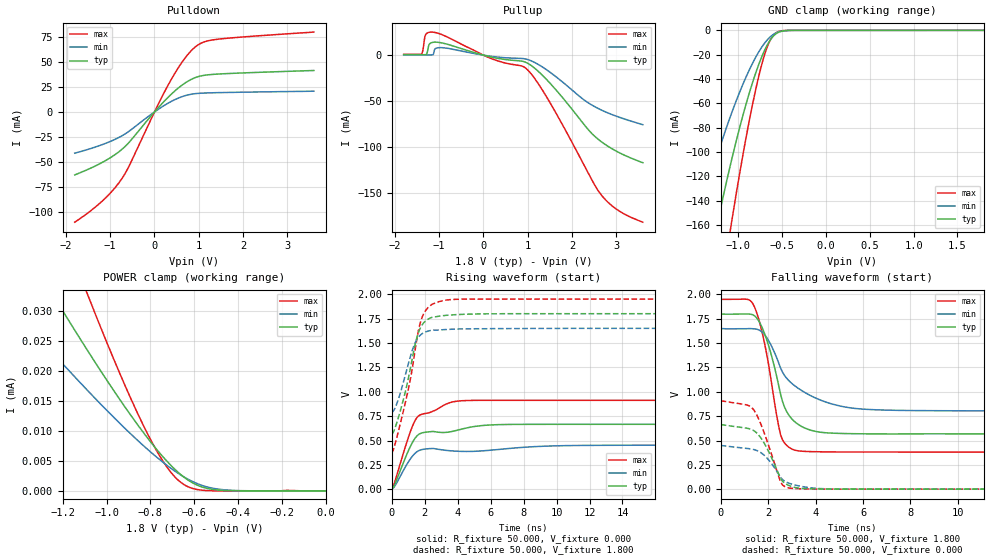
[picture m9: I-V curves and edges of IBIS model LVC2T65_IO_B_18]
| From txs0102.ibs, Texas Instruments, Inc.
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[Model]   LVC2T65_IO_B_18
Model_type  I/O
Vinl=0.15
Vinh=1.25
Enable   Active-High
Vref =   1.8V
Rref =   1000000
Cref =   15p
Vmeas =   0.9
| variable   typ   min   max
C_comp   7.28pF   6.26pF   7.93pF
| C_pullup   7.12pF   6.34pF   8.49pF
| C_pulldown   8.27pF   6.85pF   9.45pF
| C_tri-state   7.28pF   6.26pF   7.93pF
[Temperature Range]   40   100   -40
| Ambient temperature   25   85   -40
[Voltage range]   1.8   1.65   1.95
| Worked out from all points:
|   slope of the pulldown table from 0 to 0.27 V, typ, clamps not added: 20.8 ohm
|   slope of the pullup table from 0 to 0.27 V, typ, clamps not added: 89.3 ohm
|   GND clamp passes 1 mA (typ) near -0.52 V on its own axis
|   rising waveform, R_fixture 50.000, V_fixture 0.000: 20-80 % time 1.07ns typ, 979ps min, 1.12ns max; typ from 0.003 V to 0.665 V
|   falling waveform, R_fixture 50.000, V_fixture 1.800: 20-80 % time 837ps typ, 1.65ns min, 689ps max; typ from 1.8 V to 0.566 V
|   rising waveform, R_fixture 50.000, V_fixture 1.800: 20-80 % time 988ps typ, 887ps min, 1.09ns max; typ from 0.566 V to 1.8 V
|   falling waveform, R_fixture 50.000, V_fixture 0.000: 20-80 % time 803ps typ, 873ps min, 786ps max; typ from 0.665 V to 0.002 V
[GND Clamp]
| LVC2T65_IO_B_18
|   Voltage   I(typ)   I(min)   I(max)
-1.8V     -375.4mA   -251.7mA   -534.8mA
-1.505V   -256mA     -168.2mA   -372.2mA
-1.455V   -236.9mA   -155.1mA   -345.5mA
-1.245V   -161.1mA   -104mA     -237.8mA
-1.085V   -109.4mA   -69.9mA    -161.9mA
-1.065V   -103.3mA   -65.96mA   -152.9mA
-910mV    -60.44mA   -38.25mA   -87.94mA
-790mV    -32.88mA   -20.73mA   -45.28mA
-690mV    -15.04mA   -9.675mA   -17.94mA
-595mV    -4.452mA   -3.158mA   -3.768mA
-435mV    -133uA     -140.9uA   -36.64uA
1.8V      221.9pA    1.807nA    42.15pA
[POWER Clamp]
| LVC2T65_IO_B_18
|   Voltage   I(typ)   I(min)   I(max)
-1.8V     67.65uA    46.37uA    105uA
-1.475V   46.79uA    32.42uA    70.89uA
-1.245V   32.66uA    22.95uA    47.81uA
-1.09V    23.55uA    16.85uA    33uA
-1.045V   21uA       15.13uA    28.85uA
-900mV    13.13uA    9.844uA    16.23uA
-820mV    9.138uA    7.145uA    10.01uA
-740mV    5.561uA    4.691uA    4.787uA
-660mV    2.669uA    2.614uA    1.382uA
-585mV    936.6nA    1.193uA    222.3nA
-495mV    158.1nA    315.9nA    13.45nA
0V        0A         0A         0A
[Pulldown]
| LVC2T65_IO_B_18
|   Voltage   I(typ)   I(min)   I(max)
-1.8V     -62.77mA   -41.14mA   -109.8mA
-1.16V    -49.87mA   -32.31mA   -88.04mA
-950mV    -44.35mA   -28.57mA   -78.6mA
-750mV    -37.89mA   -24.23mA   -67.42mA
-575mV    -30.5mA    -19.34mA   -54.13mA
35mV      1.607mA    980.9uA    2.933mA
355mV     16.51mA    9.772mA    30.32mA
665mV     27.92mA    15.73mA    52.05mA
940mV     34.37mA    18.2mA     65.23mA
1.13V     36.41mA    18.73mA    69.74mA
1.455V    37.68mA    19.14mA    72.43mA
3.6V      41.17mA    20.55mA    79.4mA
[Pullup]
| LVC2T65_IO_B_18
|   Voltage   I(typ)   I(min)   I(max)
-1.8V     498.7uA    245.1uA    961uA
-1.395V   487.4uA    239.5uA    1.376mA
-1.305V   513.2uA    237.4uA    22.18mA
-1.225V   11.59mA    235.4uA    24.83mA
-1.135V   13.99mA    587.7uA    24.97mA
-1.08V    14.15mA    7.254mA    24.52mA
-925mV    13.2mA     8.13mA     22.11mA
150mV     -1.808mA   -1.097mA   -3.195mA
925mV     -7.183mA   -3.91mA    -13.08mA
1.415V    -25.86mA   -15.49mA   -44.39mA
2.675V    -94.48mA   -59.88mA   -152.7mA
3.6V      -116.9mA   -75.54mA   -181.5mA
[Ramp]
| LVC2T65_IO_B_18
| variable   typ   min   max
dV/dt_r   0.43/1.07E-09   0.29/9.87E-10   0.58/1.13E-09
dV/dt_f   0.73/8.35E-10   0.49/1.65E-09   0.94/6.86E-10
R_load = 50
[Rising Waveform]
R_fixture = 50.000
V_fixture = 0.000
V_fixture_min = 0.000
V_fixture_max = 0.000
C_fixture = 0.000
L_fixture = 0.000
|  time   V(typ)   V(min)   V(max)
0s        2.79mV     2.781mV    2.705mV
168ps     44.99mV    29.35mV    68.73mV
1.176ns   455.6mV    323.4mV    612.8mV
1.596ns   558.2mV    393.1mV    748.4mV
2.52ns    593.8mV    419.6mV    803.2mV
3.528ns   589.7mV    396.4mV    888.7mV
4.956ns   643.1mV    390.2mV    912.1mV
9.324ns   667mV      443.2mV    912.8mV
14.95ns   667mV      452.7mV    912.7mV
419.9ns   665.1mV    451.2mV    909mV
[Falling Waveform]
R_fixture = 50.000
V_fixture = 1.800
V_fixture_min = 1.650
V_fixture_max = 1.950
C_fixture = 0.000
L_fixture = 0.000
|  time   V(typ)   V(min)   V(max)
0s        1.799V     1.649V     1.95V
1.428ns   1.778V     1.645V     1.868V
1.932ns   1.539V     1.558V     1.395V
2.436ns   1.074V     1.301V     657.8mV
2.688ns   845mV      1.168V     475.5mV
3.276ns   664.2mV    1.034V     394.6mV
4.2ns     585.7mV    915.4mV    385mV
6.048ns   569.2mV    821.5mV    382.6mV
11.09ns   568mV      804.8mV    382.4mV
419.9ns   566.4mV    790.8mV    381.8mV
[Rising Waveform]
R_fixture = 50.000
V_fixture = 1.800
V_fixture_min = 1.650
V_fixture_max = 1.950
C_fixture = 0.000
L_fixture = 0.000
|  time   V(typ)   V(min)   V(max)
0s        566mV      790.1mV    371mV
336ps     699.1mV    891.2mV    551.2mV
924ps     1.072V     1.234V     961.8mV
1.176ns   1.28V      1.386V     1.169V
1.512ns   1.548V     1.533V     1.529V
1.68ns    1.634V     1.571V     1.674V
1.848ns   1.687V     1.596V     1.766V
2.436ns   1.762V     1.63V      1.895V
3.948ns   1.791V     1.643V     1.948V
419.9ns   1.8V       1.65V      1.95V
[Falling Waveform]
R_fixture = 50.000
V_fixture = 0.000
V_fixture_min = 0.000
V_fixture_max = 0.000
C_fixture = 0.000
L_fixture = 0.000
|  time   V(typ)   V(min)   V(max)
0s        664.7mV    450.6mV    908.7mV
1.092ns   626.9mV    419.6mV    865.3mV
1.428ns   596.5mV    405.9mV    802.3mV
1.596ns   558.2mV    390mV      724.5mV
1.848ns   467.7mV    346.3mV    568.8mV
2.52ns    113.7mV    123.9mV    76.91mV
2.604ns   83.33mV    100.3mV    46.21mV
3.108ns   20.84mV    46.16mV    8.804mV
3.864ns   5.573mV    14.2mV     3.639mV
419.9ns   2.361mV    2.039mV    2.585mV
